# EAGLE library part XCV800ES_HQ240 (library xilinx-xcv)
xcv800es_hq240 edit this description Auto generated by make-symbol-device-package-bsdl.ulp Rev. 26 Source: xcv800es_hq240.bsd
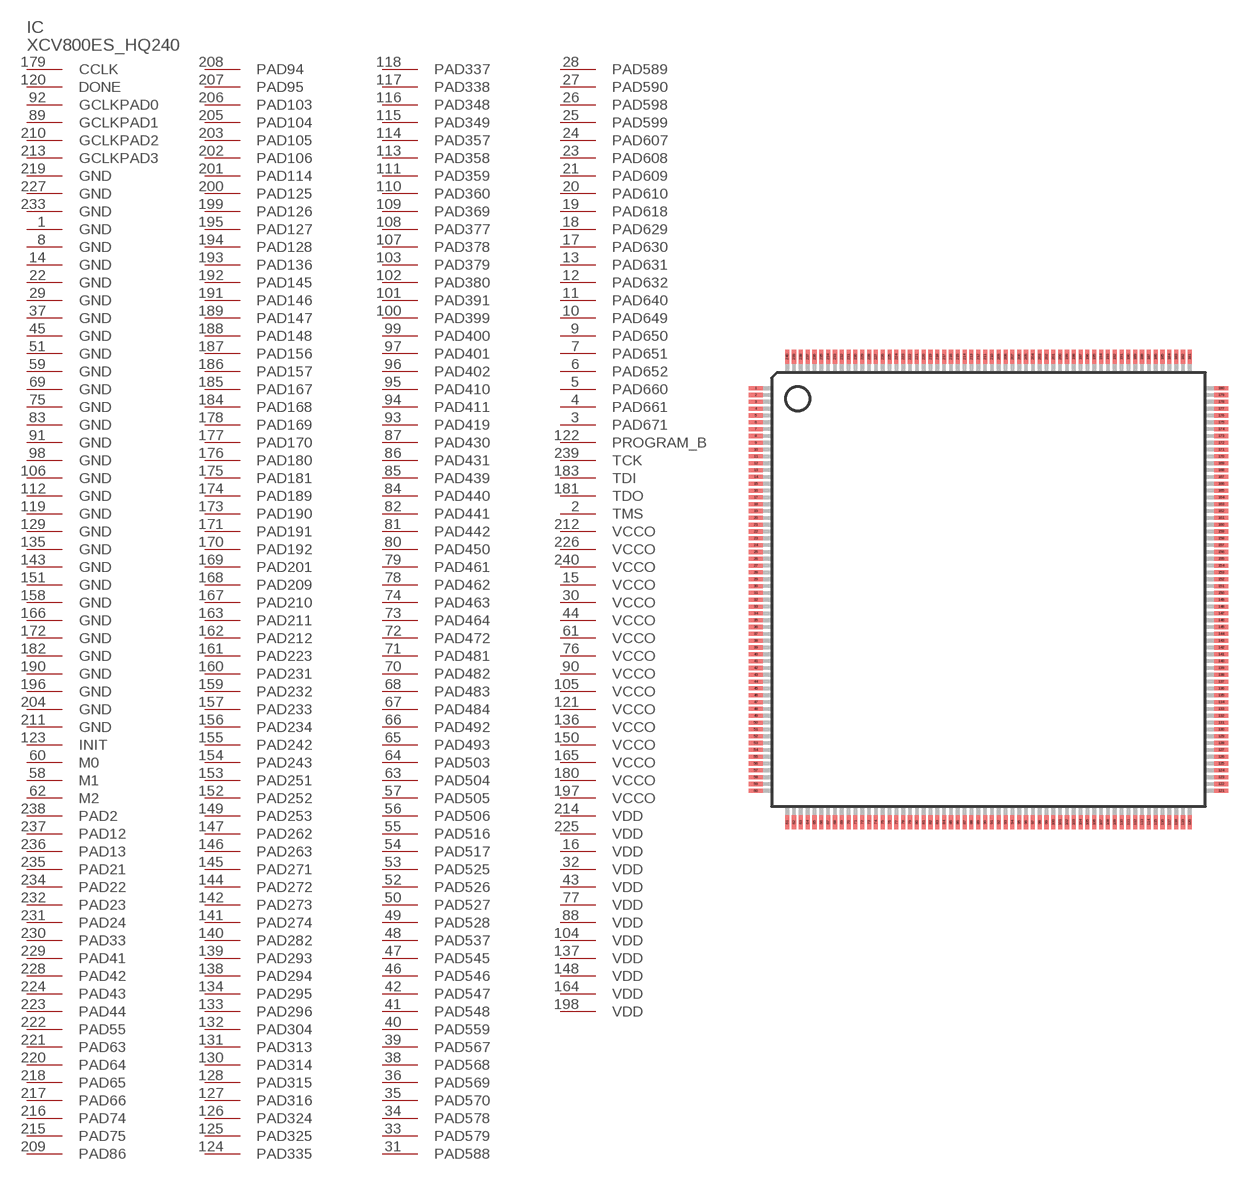
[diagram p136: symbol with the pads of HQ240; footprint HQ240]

Designator prefix IC

## XCV800ES_HQ240 (OC_FARNELL: unknown; OC_NEWARK: unknown)  [HQ240]
1  GND  pwr
2  TMS  in
3  PAD671
4  PAD661
5  PAD660
6  PAD652
7  PAD651
8  GND  pwr
9  PAD650
10  PAD649
11  PAD640
12  PAD632
13  PAD631
14  GND  pwr
15  VCCO  pwr
16  VDD  pwr
17  PAD630
18  PAD629
19  PAD618
20  PAD610
21  PAD609
22  GND  pwr
23  PAD608
24  PAD607
25  PAD599
26  PAD598
27  PAD590
28  PAD589
29  GND  pwr
30  VCCO  pwr
31  PAD588
32  VDD  pwr
33  PAD579
34  PAD578
35  PAD570
36  PAD569
37  GND  pwr
38  PAD568
39  PAD567
40  PAD559
41  PAD548
42  PAD547
43  VDD  pwr
44  VCCO  pwr
45  GND  pwr
46  PAD546
47  PAD545
48  PAD537
49  PAD528
50  PAD527
51  GND  pwr
52  PAD526
53  PAD525
54  PAD517
55  PAD516
56  PAD506
57  PAD505
58  M1  in
59  GND  pwr
60  M0  in
61  VCCO  pwr
62  M2  in
63  PAD504
64  PAD503
65  PAD493
66  PAD492
67  PAD484
68  PAD483
69  GND  pwr
70  PAD482
71  PAD481
72  PAD472
73  PAD464
74  PAD463
75  GND  pwr
76  VCCO  pwr
77  VDD  pwr
78  PAD462
79  PAD461
80  PAD450
81  PAD442
82  PAD441
83  GND  pwr
84  PAD440
85  PAD439
86  PAD431
87  PAD430
88  VDD  pwr
89  GCLKPAD1  in
90  VCCO  pwr
91  GND  pwr
92  GCLKPAD0  in
93  PAD419
94  PAD411
95  PAD410
96  PAD402
97  PAD401
98  GND  pwr
99  PAD400
100  PAD399
101  PAD391
102  PAD380
103  PAD379
104  VDD  pwr
105  VCCO  pwr
106  GND  pwr
107  PAD378
108  PAD377
109  PAD369
110  PAD360
111  PAD359
112  GND  pwr
113  PAD358
114  PAD357
115  PAD349
116  PAD348
117  PAD338
118  PAD337
119  GND  pwr
120  DONE
121  VCCO  pwr
122  PROGRAM_B  in
123  INIT
124  PAD335
125  PAD325
126  PAD324
127  PAD316
128  PAD315
129  GND  pwr
130  PAD314
131  PAD313
132  PAD304
133  PAD296
134  PAD295
135  GND  pwr
136  VCCO  pwr
137  VDD  pwr
138  PAD294
139  PAD293
140  PAD282
141  PAD274
142  PAD273
143  GND  pwr
144  PAD272
145  PAD271
146  PAD263
147  PAD262
148  VDD  pwr
149  PAD253
150  VCCO  pwr
151  GND  pwr
152  PAD252
153  PAD251
154  PAD243
155  PAD242
156  PAD234
157  PAD233
158  GND  pwr
159  PAD232
160  PAD231
161  PAD223
162  PAD212
163  PAD211
164  VDD  pwr
165  VCCO  pwr
166  GND  pwr
167  PAD210
168  PAD209
169  PAD201
170  PAD192
171  PAD191
172  GND  pwr
173  PAD190
174  PAD189
175  PAD181
176  PAD180
177  PAD170
178  PAD169
179  CCLK
180  VCCO  pwr
181  TDO  out
182  GND  pwr
183  TDI  in
184  PAD168
185  PAD167
186  PAD157
187  PAD156
188  PAD148
189  PAD147
190  GND  pwr
191  PAD146
192  PAD145
193  PAD136
194  PAD128
195  PAD127
196  GND  pwr
197  VCCO  pwr
198  VDD  pwr
199  PAD126
200  PAD125
201  PAD114
202  PAD106
203  PAD105
204  GND  pwr
205  PAD104
206  PAD103
207  PAD95
208  PAD94
209  PAD86
210  GCLKPAD2  in
211  GND  pwr
212  VCCO  pwr
213  GCLKPAD3  in
214  VDD  pwr
215  PAD75
216  PAD74
217  PAD66
218  PAD65
219  GND  pwr
220  PAD64
221  PAD63
222  PAD55
223  PAD44
224  PAD43
225  VDD  pwr
226  VCCO  pwr
227  GND  pwr
228  PAD42
229  PAD41
230  PAD33
231  PAD24
232  PAD23
233  GND  pwr
234  PAD22
235  PAD21
236  PAD13
237  PAD12
238  PAD2
239  TCK  in
240  VCCO  pwr

## Footprint HQ240 (pad centres in mm)
HQ240 Auto generated by make-symbol-device-package-bsdl.ulp Rev. 26
smd 1 x 0.3: 1 -17.05,14.75; 2 -17.05,14.25; 3 -17.05,13.75; 4 -17.05,13.25; 5 -17.05,12.75; 6 -17.05,12.25; 7 -17.05,11.75; 8 -17.05,11.25; 9 -17.05,10.75; 10 -17.05,10.25; 11 -17.05,9.75; 12 -17.05,9.25; 13 -17.05,8.75; 14 -17.05,8.25; 15 -17.05,7.75; 16 -17.05,7.25; 17 -17.05,6.75; 18 -17.05,6.25; 19 -17.05,5.75; 20 -17.05,5.25; 21 -17.05,4.75; 22 -17.05,4.25; 23 -17.05,3.75; 24 -17.05,3.25; 25 -17.05,2.75; 26 -17.05,2.25; 27 -17.05,1.75; 28 -17.05,1.25; 29 -17.05,0.75; 30 -17.05,0.25; 31 -17.05,-0.25; 32 -17.05,-0.75; 33 -17.05,-1.25; 34 -17.05,-1.75; 35 -17.05,-2.25; 36 -17.05,-2.75; 37 -17.05,-3.25; 38 -17.05,-3.75; 39 -17.05,-4.25; 40 -17.05,-4.75; 41 -17.05,-5.25; 42 -17.05,-5.75; 43 -17.05,-6.25; 44 -17.05,-6.75; 45 -17.05,-7.25; 46 -17.05,-7.75; 47 -17.05,-8.25; 48 -17.05,-8.75; 49 -17.05,-9.25; 50 -17.05,-9.75; 51 -17.05,-10.25; 52 -17.05,-10.75; 53 -17.05,-11.25; 54 -17.05,-11.75; 55 -17.05,-12.25; 56 -17.05,-12.75; 57 -17.05,-13.25; 58 -17.05,-13.75; 59 -17.05,-14.25; 60 -17.05,-14.75; 121 17.05,-14.75; 122 17.05,-14.25; 123 17.05,-13.75; 124 17.05,-13.25; 125 17.05,-12.75; 126 17.05,-12.25; 127 17.05,-11.75; 128 17.05,-11.25; 129 17.05,-10.75; 130 17.05,-10.25; 131 17.05,-9.75; 132 17.05,-9.25; 133 17.05,-8.75; 134 17.05,-8.25; 135 17.05,-7.75; 136 17.05,-7.25; 137 17.05,-6.75; 138 17.05,-6.25; 139 17.05,-5.75; 140 17.05,-5.25; 141 17.05,-4.75; 142 17.05,-4.25; 143 17.05,-3.75; 144 17.05,-3.25; 145 17.05,-2.75; 146 17.05,-2.25; 147 17.05,-1.75; 148 17.05,-1.25; 149 17.05,-0.75; 150 17.05,-0.25; 151 17.05,0.25; 152 17.05,0.75; 153 17.05,1.25; 154 17.05,1.75; 155 17.05,2.25; 156 17.05,2.75; 157 17.05,3.25; 158 17.05,3.75; 159 17.05,4.25; 160 17.05,4.75; 161 17.05,5.25; 162 17.05,5.75; 163 17.05,6.25; 164 17.05,6.75; 165 17.05,7.25; 166 17.05,7.75; 167 17.05,8.25; 168 17.05,8.75; 169 17.05,9.25; 170 17.05,9.75; 171 17.05,10.25; 172 17.05,10.75; 173 17.05,11.25; 174 17.05,11.75; 175 17.05,12.25; 176 17.05,12.75; 177 17.05,13.25; 178 17.05,13.75; 179 17.05,14.25; 180 17.05,14.75
smd 0.3 x 1: 61 -14.75,-17.05; 62 -14.25,-17.05; 63 -13.75,-17.05; 64 -13.25,-17.05; 65 -12.75,-17.05; 66 -12.25,-17.05; 67 -11.75,-17.05; 68 -11.25,-17.05; 69 -10.75,-17.05; 70 -10.25,-17.05; 71 -9.75,-17.05; 72 -9.25,-17.05; 73 -8.75,-17.05; 74 -8.25,-17.05; 75 -7.75,-17.05; 76 -7.25,-17.05; 77 -6.75,-17.05; 78 -6.25,-17.05; 79 -5.75,-17.05; 80 -5.25,-17.05; 81 -4.75,-17.05; 82 -4.25,-17.05; 83 -3.75,-17.05; 84 -3.25,-17.05; 85 -2.75,-17.05; 86 -2.25,-17.05; 87 -1.75,-17.05; 88 -1.25,-17.05; 89 -0.75,-17.05; 90 -0.25,-17.05; 91 0.25,-17.05; 92 0.75,-17.05; 93 1.25,-17.05; 94 1.75,-17.05; 95 2.25,-17.05; 96 2.75,-17.05; 97 3.25,-17.05; 98 3.75,-17.05; 99 4.25,-17.05; 100 4.75,-17.05; 101 5.25,-17.05; 102 5.75,-17.05; 103 6.25,-17.05; 104 6.75,-17.05; 105 7.25,-17.05; 106 7.75,-17.05; 107 8.25,-17.05; 108 8.75,-17.05; 109 9.25,-17.05; 110 9.75,-17.05; 111 10.25,-17.05; 112 10.75,-17.05; 113 11.25,-17.05; 114 11.75,-17.05; 115 12.25,-17.05; 116 12.75,-17.05; 117 13.25,-17.05; 118 13.75,-17.05; 119 14.25,-17.05; 120 14.75,-17.05; 181 14.75,17.05; 182 14.25,17.05; 183 13.75,17.05; 184 13.25,17.05; 185 12.75,17.05; 186 12.25,17.05; 187 11.75,17.05; 188 11.25,17.05; 189 10.75,17.05; 190 10.25,17.05; 191 9.75,17.05; 192 9.25,17.05; 193 8.75,17.05; 194 8.25,17.05; 195 7.75,17.05; 196 7.25,17.05; 197 6.75,17.05; 198 6.25,17.05; 199 5.75,17.05; 200 5.25,17.05; 201 4.75,17.05; 202 4.25,17.05; 203 3.75,17.05; 204 3.25,17.05; 205 2.75,17.05; 206 2.25,17.05; 207 1.75,17.05; 208 1.25,17.05; 209 0.75,17.05; 210 0.25,17.05; 211 -0.25,17.05; 212 -0.75,17.05; 213 -1.25,17.05; 214 -1.75,17.05; 215 -2.25,17.05; 216 -2.75,17.05; 217 -3.25,17.05; 218 -3.75,17.05; 219 -4.25,17.05; 220 -4.75,17.05; 221 -5.25,17.05; 222 -5.75,17.05; 223 -6.25,17.05; 224 -6.75,17.05; 225 -7.25,17.05; 226 -7.75,17.05; 227 -8.25,17.05; 228 -8.75,17.05; 229 -9.25,17.05; 230 -9.75,17.05; 231 -10.25,17.05; 232 -10.75,17.05; 233 -11.25,17.05; 234 -11.75,17.05; 235 -12.25,17.05; 236 -12.75,17.05; 237 -13.25,17.05; 238 -13.75,17.05; 239 -14.25,17.05; 240 -14.75,17.05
